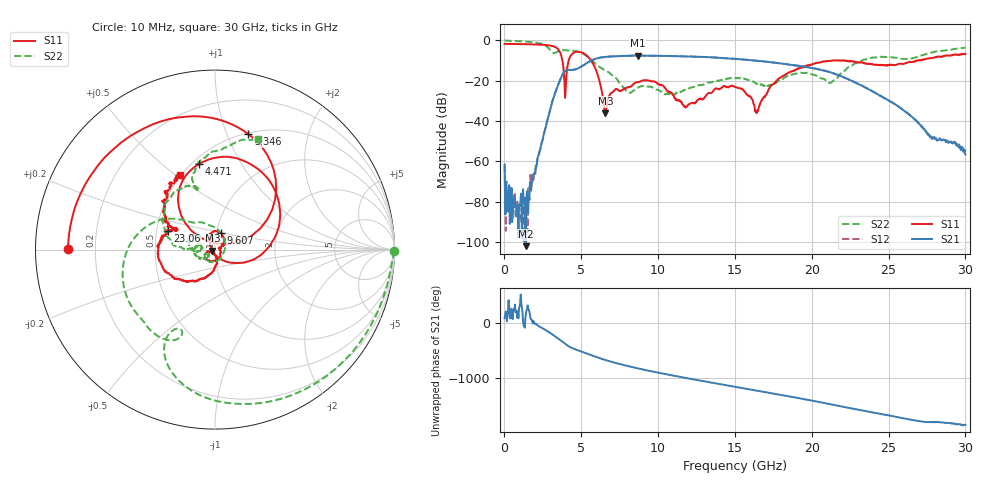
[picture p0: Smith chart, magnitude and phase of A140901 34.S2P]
!  2-Port S-parameters saved by WinCal
! VAR MeasName=S-Parameters (CALIBRATED_DATA) read from VNA (N5244A)
! VAR MeasDate=11/3/2014 9:33:10 AM
! VAR NAME=A140901 34
! VAR FILENAME=A140901 34.S2P
! VAR DATE=11/3/2014 9:33:10 AM
! VAR PHYS_PORTS=1,2
# Hz S RI R 50
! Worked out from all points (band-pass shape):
!   801 points, 10 MHz to 30 GHz, reference 50 ohm
!   highest |S21| = -7.51 dB at 8.67 GHz (marker M1); lowest = -102.0 dB at 1.397 GHz (marker M2)
!   |S21| within 3 dB of the highest: 5.522 GHz to 16.98 GHz (11.46 GHz wide, 102 % of centre)
!   lowest |S11| = -36.1 dB at 6.57 GHz (marker M3), VSWR 1.03, Z = 48.6 - j0.658 ohm
!   |S11| at or under -10 dB: 3.77 GHz to 4.178 GHz (408.2 MHz wide, 10.3 % of centre); 5.637 GHz to 21.36 GHz (15.72 GHz wide, 116 % of centre); 22.12 GHz to 26.84 GHz (4.725 GHz wide, 19.3 % of centre)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
!   |S22| runs from -27.4 to 0.0 dB; largest |S21 - S12| = 0.0029
!   S11 on the Smith chart (normalised r, x): 10 MHz: 0.10, +0.00; 3.346 GHz: 0.51, +1.19; 4.471 GHz: 0.54, +0.67; 9.607 GHz: 1.05, +0.19; 23.06 GHz: 0.58, +0.13; 30 GHz: 0.49, +0.52
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1e7  -0.8185 0.00278  1.63e-06 0.000838  -0.00078 -0.000268  0.9971 -0.00862
3.473875e8  -0.8087 0.1133  -2.01e-05 2.01e-05  -0.000104 0.000138  0.952 -0.2216
1.397038e9  -0.6772 0.4338  -7.88e-06 1.09e-06  7.11e-05 -9.76e-05  0.5801 -0.7333
3.346388e9  0.1853 0.6438  -0.0177 0.0532  -0.0178 0.0531  -0.1828 -0.468
3.946188e9  0.0202 0.0318  0.1656 -0.0521  0.1653 -0.0515  -0.3749 -0.4315
4.471012e9  -0.0912 0.476  -0.0459 -0.181  -0.0451 -0.1803  -0.4903 -0.2644
5.033325e9  0.2768 0.4149  -0.2179 -0.0673  -0.2177 -0.0681  -0.4866 0.00136
5.895538e9  0.2016 -0.0606  -0.1137 0.3271  -0.115 0.3275  -0.2072 0.1703
6.570312e9  -0.0142 -0.00676  0.2728 0.2772  0.2729 0.2772  -0.0962 0.1509
8.669612e9  -0.0264 0.0888  -0.1238 -0.4024  -0.1236 -0.4016  0.00242 -0.066
9.6068e9  0.034 0.0912  -0.3983 -0.1173  -0.3966 -0.1178  -0.0565 -0.0414
1.001916e10  0.0473 0.0673  -0.4121 0.0497  -0.4104 0.0489  -0.054 -0.026
1.181856e10  0.0222 0.00506  0.095 0.3899  0.0957 0.3897  -0.0413 -0.0434
1.331806e10  0.0302 -0.0397  0.3842 -0.00531  0.3842 -0.00517  -0.0748 -0.0522
1.5005e10  -0.0539 -0.045  0.0295 -0.347  0.0291 -0.3472  -0.1157 -0.00976
1.642952e10  -0.0122 -0.0101  -0.2844 -0.1274  -0.285 -0.1287  -0.0798 0.0232
1.785405e10  -0.00391 -0.1126  -0.1858 0.1992  -0.1869 0.1988  -0.1007 -0.0133
2.002832e10  -0.1932 -0.1662  0.1921 0.0759  0.1928 0.0765  -0.115 0.0831
2.122792e10  -0.2997 -0.074  0.1146 -0.1135  0.1146 -0.1131  -0.0816 0.0389
2.306481e10  -0.2611 0.102  -0.0684 -0.0457  -0.0681 -0.0463  -0.2789 0.1005
2.501416e10  -0.212 0.1144  -0.0116 0.0302  -0.0119 0.0301  -0.1602 0.3554
3e10  -0.1969 0.4175  0.000649 -0.00134  0.000637 -0.00186  0.2375 0.6177
